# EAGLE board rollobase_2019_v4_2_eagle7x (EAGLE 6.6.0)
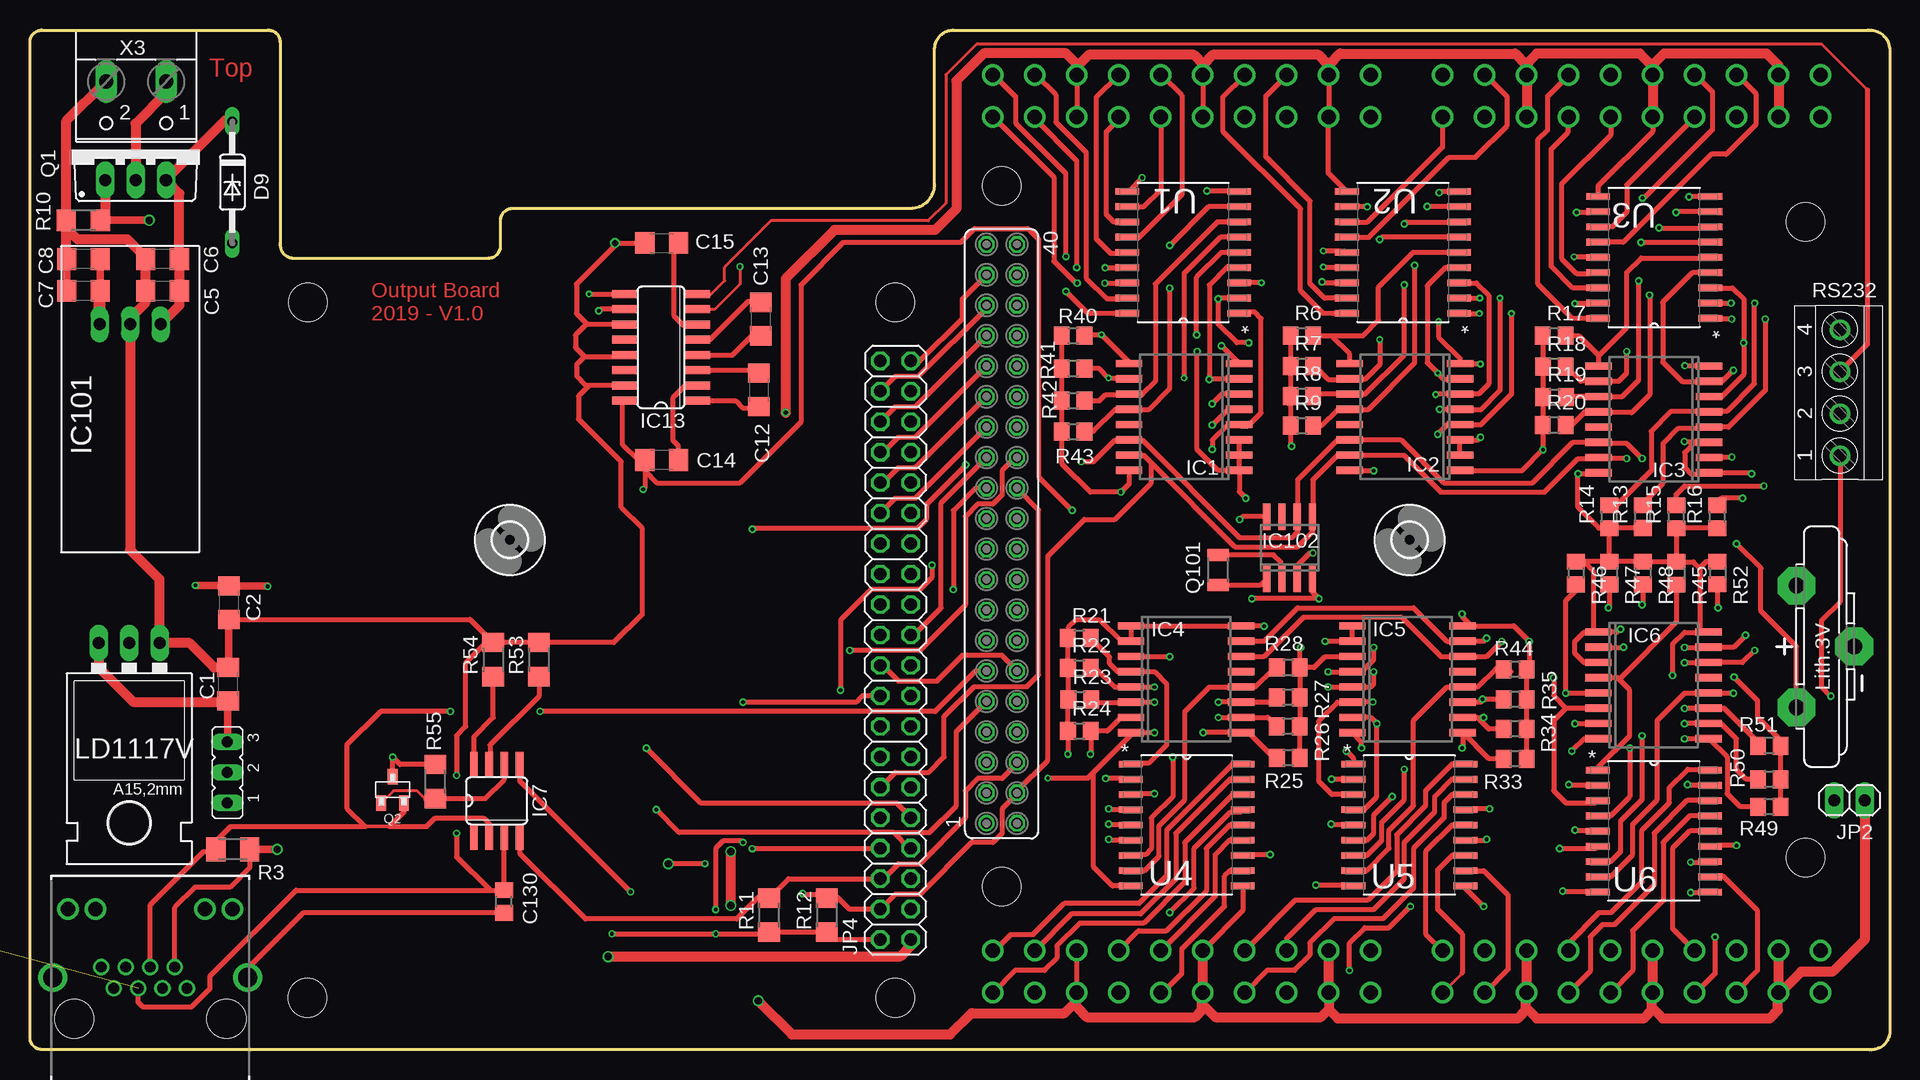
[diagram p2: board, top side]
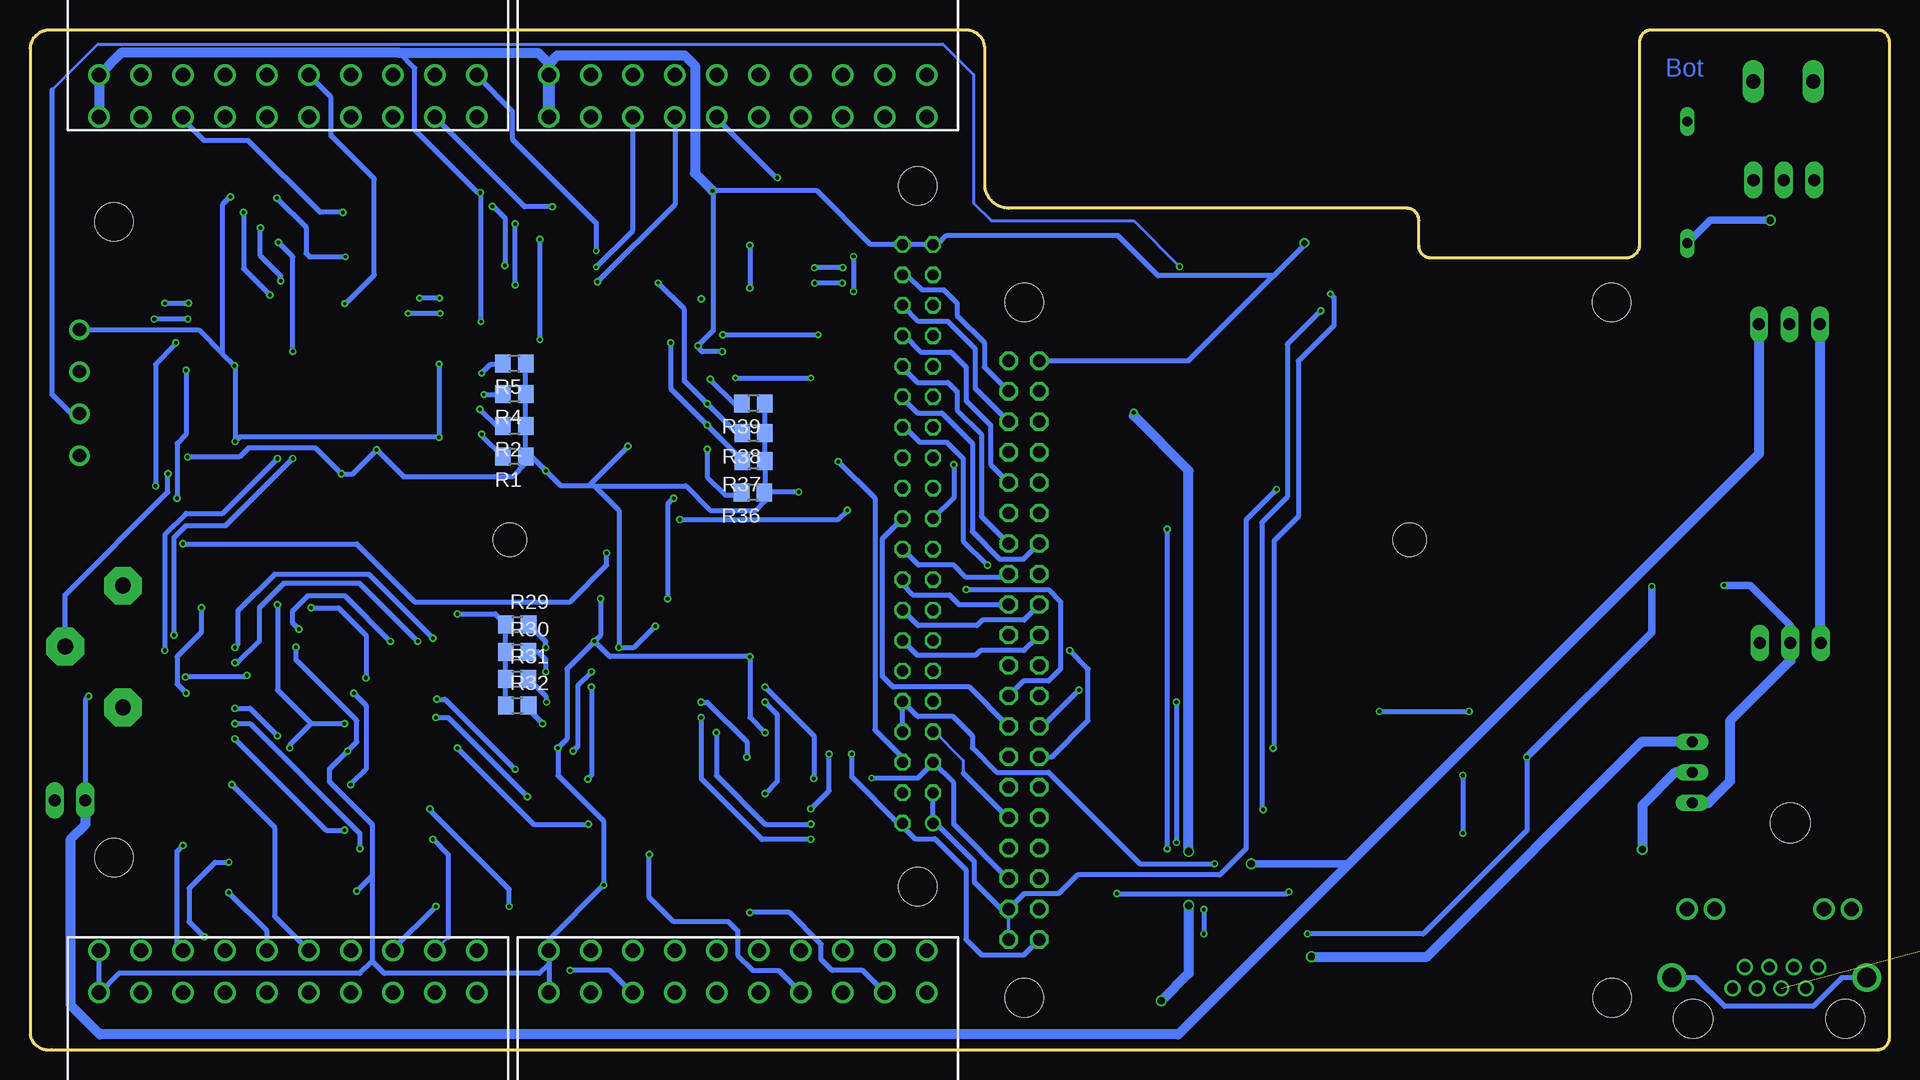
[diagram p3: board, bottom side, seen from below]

Size 155 x 85.03 mm. Coordinates in mm from the lower left corner, seen from the top.
Outline: 153.2,0.02 1,0.02 arc-90 0,1.02 0,84.02 arc-90 1,85.02 19.85,85.02 arc-90 20.85,84.02 20.85,67.27 arc90 21.85,66.02 38.23,66.02 arc90 39.23,67.02 39.23,69.17 arc-90 40.23,70.17 73.42,70.17 arc90 75.42,72.17 75.42,83.52 arc-90 77.02,85.02 153.2,85.02 arc-90 155,83.52 155,1.29 arc-90 153.2,0.02
Copper layers (1*16): Top 0.035mm / dielectric 1.6mm / Bottom 0.035mm
Design rules "JLCPCB_2-layer_PCB_eagle_rule": minimum track width 3.5mil, minimum drill 0.2mm, track to track 6mil, track to pad 6mil, pad to pad 6mil, via to via 8mil, smd to smd 0mil, copper to edge 20mil, drill to drill 10mil, minimum pad ring 6mil, minimum via ring 6mil, stop-mask expansion 0mil, vias tented up to drill 100mil, thermal gap 10mil
Net classes: 0 default: clearance 0.203 mm; 1 signal: width 0.406 mm, drill 0.254 mm, clearance 0.203 mm
Holes 3.2 mm at 23.16,62.33 72.11,62.33 72.14,4.34 81,72.02 81,13.62 148.02,16.02 23.13,4.34 148.02,69.02

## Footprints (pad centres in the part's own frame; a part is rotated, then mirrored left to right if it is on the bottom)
CR2032V = drill 1.321 pad 3.15 octagon: + -2.54,-5.08; +@1 -2.54,5.08; - 2.286,0
C1206 = smd 1.6 x 1.8: 1 -1.4,0; 2 1.4,0
R0805 = smd 1.3 x 1.5: 1 -0.95,0; 2 0.95,0
DO35Z10 = drill 0.813 long: A 5.08,0; C -5.08,0
SO16W = smd 0.6 x 2.2: 1 -4.445,-4.6; 2 -3.175,-4.6; 3 -1.905,-4.6; 4 -0.635,-4.6; 5 0.635,-4.6; 6 1.905,-4.6; 7 3.175,-4.6; 8 4.445,-4.6; 9 4.445,4.6; 10 3.175,4.6; 11 1.905,4.6; 12 0.635,4.6; 13 -0.635,4.6; 14 -1.905,4.6; 15 -3.175,4.6; 16 -4.445,4.6
SO08 = smd 0.66 x 2.032: 1 -1.905,-3.073; 2 -0.635,-3.073; 3 0.635,-3.073; 4 1.905,-3.073; 5 1.905,3.073; 6 0.635,3.073; 7 -0.635,3.073; 8 -1.905,3.073
SO16 = smd 0.66 x 2.032: 1 -4.445,-3.073; 2 -3.175,-3.073; 3 -1.905,-3.073; 4 -0.635,-3.073; 5 0.635,-3.073; 6 1.905,-3.073; 7 3.175,-3.073; 8 4.445,-3.073; 9 4.445,3.073; 10 3.175,3.073; 11 1.905,3.073; 12 0.635,3.073; 13 -0.635,3.073; 14 -1.905,3.073; 15 -3.175,3.073; 16 -4.445,3.073
SIP3 = drill 1 long: 1 -2.54,0; 2 0,0; 3 2.54,0
SO08' = smd 0.6 x 2.2: 1 -1.905,-2.6; 2 -0.635,-2.6; 3 0.635,-2.6; 4 1.905,-2.6; 5 1.905,2.6; 6 0.635,2.6; 7 -0.635,2.6; 8 -1.905,2.6
0569564 = drill 0.9: 1 -4.445,6.35; 2 -3.175,8.89; 3 -1.905,6.35; 4 -0.635,8.89; 5 0.635,6.35; 6 1.905,8.89; 7 3.175,6.35; 8 4.445,8.89 | drill 1.2: A1 -6.295,-4.32; A2 3.835,-4.32; C1 -3.755,-2.79; C2 6.375,-2.79 | drill 1.6: S1 -7.745,3.05; S2 7.745,3.05 | hole 3.25: -5.715,0; 5.715,0
0569564' = drill 0.9: 1 3.06,-0.89; 2 2.04,0.89; 3 1.02,-0.89; 4 0,0.89; 5 -1.02,-0.89; 6 -2.04,0.89; 7 -3.06,-0.89; 8 -4.08,0.89 | drill 1.2: A1 -6.86,5.71; A2 4.57,5.71; C1 -4.57,5.71; C2 6.86,5.71 | drill 1.6: S1 8.125,0; S2 -8.125,0 | hole 3.25: -6.35,-3.43; 6.35,-3.43
FE20-2 = drill 0.914: 1 -24.13,1.27 | drill 0.914 octagon: 2 -24.13,-1.27; 3 -21.59,1.27; 4 -21.59,-1.27; 5 -19.05,1.27; 6 -19.05,-1.27; 7 -16.51,1.27; 8 -16.51,-1.27; 9 -13.97,1.27; 10 -13.97,-1.27; 11 -11.43,1.27; 12 -11.43,-1.27; 13 -8.89,1.27; 14 -8.89,-1.27; 15 -6.35,1.27; 16 -6.35,-1.27; 17 -3.81,1.27; 18 -3.81,-1.27; 19 -1.27,1.27; 20 -1.27,-1.27; 21 1.27,1.27; 22 1.27,-1.27; 23 3.81,1.27; 24 3.81,-1.27; 25 6.35,1.27; 26 6.35,-1.27; 27 8.89,1.27; 28 8.89,-1.27; 29 11.43,1.27; 30 11.43,-1.27; 31 13.97,1.27; 32 13.97,-1.27; 33 16.51,1.27; 34 16.51,-1.27; 35 19.05,1.27; 36 19.05,-1.27; 37 21.59,1.27; 38 21.59,-1.27; 39 24.13,1.27; 40 24.13,-1.27
1X02 = drill 1.016 long: 1 -1.27,0; 2 1.27,0
2X20 = drill 1.016 octagon: 1 -24.13,-1.27; 2 -24.13,1.27; 3 -21.59,-1.27; 4 -21.59,1.27; 5 -19.05,-1.27; 6 -19.05,1.27; 7 -16.51,-1.27; 8 -16.51,1.27; 9 -13.97,-1.27; 10 -13.97,1.27; 11 -11.43,-1.27; 12 -11.43,1.27; 13 -8.89,-1.27; 14 -8.89,1.27; 15 -6.35,-1.27; 16 -6.35,1.27; 17 -3.81,-1.27; 18 -3.81,1.27; 19 -1.27,-1.27; 20 -1.27,1.27; 21 1.27,-1.27; 22 1.27,1.27; 23 3.81,-1.27; 24 3.81,1.27; 25 6.35,-1.27; 26 6.35,1.27; 27 8.89,-1.27; 28 8.89,1.27; 29 11.43,-1.27; 30 11.43,1.27; 31 13.97,-1.27; 32 13.97,1.27; 33 16.51,-1.27; 34 16.51,1.27; 35 19.05,-1.27; 36 19.05,1.27; 37 21.59,-1.27; 38 21.59,1.27; 39 24.13,-1.27; 40 24.13,1.27
78XXL = drill 1.016 long: GND 0,-3.81; IN -2.54,-3.81; OUT 2.54,-3.81 | hole 3.302: 0,11.176
JP2 = drill 0.914 long: 1 -2.54,0; 2 0,0; 3 2.54,0
713-1425 = drill 1.2: 1 -15.75,-1.75; 2 -15.75,1.75; 3 -12.25,-1.75; 4 -12.25,1.75; 5 -8.75,-1.75; 6 -8.75,1.75; 7 -5.25,-1.75; 8 -5.25,1.75; 9 -1.75,-1.75; 10 -1.75,1.75; 11 1.75,-1.75; 12 1.75,1.75; 13 5.25,-1.75; 14 5.25,1.75; 15 8.75,-1.75; 16 8.75,1.75; 17 12.25,-1.75; 18 12.25,1.75; 19 15.75,-1.75; 20 15.75,1.75
TO220BV = drill 1.016 long: D 0,-2.54; G -2.54,-2.54; S 2.54,-2.54
SOT23 = smd 1.3 x 0.9: 1 -1.1,0.95; 2 -1.1,-0.95; 3 1.1,0
QSMD = smd 1 x 1.8: 1 -1.25,0; 2 1.25,0
M1206 = smd 1.6 x 2: 1 -1.4,0; 2 1.4,0
R1206 = smd 1.6 x 1.803: 1 -1.422,0; 2 1.422,0
TERMINAL-BLOCK-4-PIN-3.5MM-ROUND-PAD = drill 1.1 pad 1.7: 1 -5.25,-0.1; 2 -1.75,-0.1; 3 1.75,-0.1; 4 5.25,-0.1
TIULN2803ADW_SOIC127P1030X265-18N = smd 1.981 x 0.559: 1 -4.674,5.08; 2 -4.674,3.81; 3 -4.674,2.54; 4 -4.674,1.27; 5 -4.674,0; 6 -4.674,-1.27; 7 -4.674,-2.54; 8 -4.674,-3.81; 9 -4.674,-5.08; 10 4.674,-5.08; 11 4.674,-3.81; 12 4.674,-2.54; 13 4.674,-1.27; 14 4.674,0; 15 4.674,1.27; 16 4.674,2.54; 17 4.674,3.81; 18 4.674,5.08
2,8 = hole 2.8: 0,0
RJ45-TRAFO-L = drill 1: 1 -4.445,6.35; 2 -3.175,8.89; 3 -1.905,6.35; 4 -0.635,8.89; 5 0.635,6.35; 6 1.905,8.89; 7 3.175,6.35; 8 4.445,8.89 | drill 1.6: GND1 -7.62,2.54; GND2 7.62,2.54 | drill 1.1: LEDG+ -6.35,-5.08; LEDG- -3.81,-5.08; LEDY+ 3.81,-5.08; LEDY- 6.35,-5.08 | hole 3.2: -5.08,0; 5.08,0
W237-102 = drill 1.194 long: 1 -2.5,-1.27; 2 2.5,-1.27

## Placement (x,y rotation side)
BAT  CR2032V  [CR2032V]  149.79,33.62 0 top
C1  1uF  [C1206]  16.52,30.48 90 top
C2  1uF  [C1206]  16.57,37.29 270 top
C5  1uF  [C1206]  11.05,63.27 180 top
C6  1uF  [C1206]  11.05,65.92 180 top
C7  1uF  [C1206]  4.45,63.27 180 top
C8  1uF  [C1206]  4.45,65.92 180 top
C12  1µF  [C1206]  60.75,55.02 270 top
C13  1µF  [C1206]  60.9,60.92 270 top
C14  1µF  [C1206]  52.65,49.17 180 top
C15  1µF  [C1206]  52.65,67.27 0 top
C130  1nF  [R0805]  39.51,12.37 90 top
D9  ZPD  [DO35Z10]  16.86,72.33 270 top
IC1  PCF8574T  [SO16W]  96.21,52.77 90 top
IC2  PCF8574T  [SO16W]  114.6,52.77 90 top
IC3  PCF8574T  [SO16W]  135.35,52.57 90 top
IC4  PCF8574T  [SO16W]  96.37,30.9 270 top
IC5  PCF8574T  [SO16W]  114.83,30.9 270 top
IC6  PCF8574T  [SO16W]  135.33,30.39 270 top
IC7  DS2482-100S  [SO08]  38.91,20.77 0 top
IC13  MAX3232CSE  [SO16]  52.6,58.57 90 top
IC101  R-78B5.0_SIP3  [SIP3]  8.34,60.49 180 top
IC102  DS1307_SO8  [SO08']  104.99,41.86 0 top
J1  0569564-2  [0569564]  not placed on the board
J103  0569564-  [0569564']  10.03,6.02 0 top
JP1  jp1  [FE20-2]  81,43.02 90 top
JP2  0  [1X02]  151.66,20.8 0 top
JP4  0  [2X20]  72.15,33.32 90 top
LD1117V  V_REG_LD1117VXX  [78XXL]  8.26,30.11 180 top
OW  0  [JP2]  16.45,23.12 90 top
P13  713-1430  [713-1425]  96,79.52 180 bottom
P14  713-1430  [713-1425]  133.5,79.51 180 bottom
P15  713-1430  [713-1425]  96,6.52 0 bottom
P16  713-1430  [713-1425]  133.5,6.52 0 bottom
Q1  IRF9530  [TO220BV]  8.8,75.06 0 top
Q2  TSM 3401 SOT-23  [SOT23]  30.23,21.69 90 top
Q101  32.768KHZ_SMD  [QSMD]  99.04,40.01 270 top
R1  1k  [R0805]  114.63,49.46 180 bottom
R2  1k  [R0805]  114.63,51.99 180 bottom
R3  2k2  [M1206]  16.9,16.72 0 top
R4  1k  [R0805]  114.63,54.68 180 bottom
R5  1k  [R0805]  114.63,57.21 180 bottom
R6  1k  [R0805]  106.02,59.55 0 top
R7  1k  [R0805]  106.02,57.02 0 top
R8  1k  [R0805]  106.02,54.49 0 top
R9  1k  [R0805]  106.02,52.06 0 top
R10  100K  [R1206]  4.45,69.16 0 top
R11  1k  [R1206]  61.6,11.24 90 top
R12  1k  [R1206]  66.41,11.24 90 top
R13  1k  [R0805]  134.44,44.46 90 top
R14  1k  [R0805]  131.65,44.45 90 top
R15  1k  [R0805]  137.23,44.45 90 top
R16  1k  [R0805]  140.65,44.45 90 top
R17  1k  [R0805]  127.04,59.54 0 top
R18  1k  [R0805]  127.06,56.98 0 top
R19  1k  [R0805]  127.09,54.43 0 top
R20  1k  [R0805]  127.04,52.1 0 top
R21  1k  [R0805]  87.46,34.33 0 top
R22  1k  [R0805]  87.47,31.85 0 top
R23  1k  [R0805]  87.51,29.21 0 top
R24  1k  [R0805]  87.47,26.58 0 top
R25  1k  [R0805]  104.89,24.35 180 top
R26  1k  [R0805]  104.88,26.97 180 top
R27  1k  [R0805]  104.89,29.38 180 top
R28  1k  [R0805]  104.89,31.87 180 top
R29  1k  [R0805]  114.39,35.47 0 bottom
R30  1k  [R0805]  114.39,33.18 0 bottom
R31  1k  [R0805]  114.4,30.92 0 bottom
R32  1k  [R0805]  114.39,28.71 0 bottom
R33  1k  [R0805]  123.79,24.27 180 top
R34  1k  [R0805]  123.79,26.76 180 top
R35  1k  [R0805]  123.79,29.23 180 top
R36  1k  [R0805]  94.74,46.46 180 bottom
R37  1k  [R0805]  94.69,49.09 180 bottom
R38  1k  [R0805]  94.69,51.41 180 bottom
R39  1k  [R0805]  94.72,53.9 180 bottom
R40  1k  [R0805]  86.95,59.55 0 top
R41  1k  [R0805]  86.95,56.82 0 top
R42  1k  [R0805]  86.95,54.13 0 top
R43  1k  [R0805]  86.95,51.55 0 top
R44  1k  [R0805]  123.79,31.71 180 top
R45  1k  [R0805]  137.24,39.73 270 top
R46  1k  [R0805]  128.86,39.75 270 top
R47  1k  [R0805]  131.65,39.75 270 top
R48  1k  [R0805]  134.44,39.75 270 top
R49  1k  [R0805]  144.98,20.27 180 top
R50  1k  [R0805]  144.98,22.55 180 top
R51  1k  [R0805]  144.98,25.35 180 top
R52  1k  [R0805]  140.66,39.76 270 top
R53  0R  [R1206]  42.42,32.53 90 top
R54  0R  [R1206]  38.61,32.53 90 top
R55  0R  [R1206]  33.78,22.37 270 top
RS232  TERMINAL-BLOCK-3.5MM -- RND 205-00102  [TERMINAL-BLOCK-4-PIN-3.5MM-ROUND-PAD]  150.77,54.79 90 top
U1  TIULN2803ADW_ULN2803ADW  [TIULN2803ADW_SOIC127P1030X265-18N]  96.12,66.48 180 top
U2  TIULN2803ADW_ULN2803ADW  [TIULN2803ADW_SOIC127P1030X265-18N]  114.45,66.48 180 top
U3  TIULN2803ADW_ULN2803ADW  [TIULN2803ADW_SOIC127P1030X265-18N]  135.38,66.07 180 top
U4  TIULN2803ADW_ULN2803ADW  [TIULN2803ADW_SOIC127P1030X265-18N]  96.42,18.75 0 top
U5  TIULN2803ADW_ULN2803ADW  [TIULN2803ADW_SOIC127P1030X265-18N]  114.97,18.75 0 top
U6  TIULN2803ADW_ULN2803ADW  [TIULN2803ADW_SOIC127P1030X265-18N]  135.37,18.24 0 top
U$1  [2,8]  40,42.52 0 top
U$2  [2,8]  115,42.52 0 top
U$3  RJ45-TRAFO-L  [RJ45-TRAFO-L]  not placed on the board
U$4  [WAGO288-001]  40.14,42.52 270 top
X3  VERSORGUNG  [W237-102]  8.85,79.46 180 top

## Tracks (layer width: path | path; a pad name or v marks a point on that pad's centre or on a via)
$N5555
  Top 0.406: J103.S1 18.15,6.79 22.79,11.42 C130.1
  Bottom 0.406: J103.S2 3.96,6.02 6.36,3.62 13.75,3.62 16.15,6.02 J103.S1
+3V3  (via drill 0.3)
  Top 0.254: 16.53,38.72 C2.1 | 67,9.19 67,9.23 | 61.46,9.67 R11.1 | v19.81,38.63 19.75,38.69
  Top 0.406: JP4.2 67,9.19 | 129.5,40.7 130.3,39.9 130.3,34.98 130.46,34.82 | IC1.16 91.61,47.18 v90.93,46.5 88.39,46.5 86,48.9 R43.1 R42.1 R41.1 R40.1 | R6.1 R7.1 R8.1 | R8.1 105.07,54.04 104.9,53.87 104.9,54.32 R8.1 | R8.1 R9.1 105.07,50.4 v105.16,50.31 | IC2.16 111.98,48.32 v112.01,48.28 | R17.1 126.09,57 R18.1 126.11,54.45 R19.1 126.14,52.15 | v105.92,33.55 105.84,33.47 R28.1 | v102.87,35.33 100.98,35.33 IC4.16 IC4.1 IC4.2 90.92,34.07 89.15,35.84 87.17,35.84 86.54,35.2 86.54,34.36 R21.1 86.52,34.32 R22.1 86.56,31.8 R23.1 86.52,29.16 R24.1 v86.52,24.67 v86.51,24.66 | R49.1 R50.1 R51.1 145.93,25.8 144.02,27.71 144.02,29.11 v142.04,31.09 | 138.94,34.82 137.92,34.82 136.91,33.8 v136.91,31.21 | 138.94,34.82 139.92,34.82 IC6.16 | R45.1 134.46,40.68 R48.1 R47.1 | R47.1 129.5,40.7 | R45.1 138.66,40.68 139.19,40.15 | 139.19,40.15 139.19,35.07 138.94,34.82 | 120.14,35.34 123.68,35.34 v124.97,34.06 124.97,31.94 R44.1 R35.1 R34.1 R33.1 | v132.59,35.07 132.51,35.07 132.27,34.83 IC6.1 130.48,34.83 130.46,34.82 | R28.1 107.03,31.87 107.95,32.79 110.21,32.79 IC5.3 | IC5.16 120.14,35.34 | 126.14,52.15 126.14,50.06 v126.11,50.04 124.4,48.32 IC2.1 | 126.14,52.15 R20.1 | 129.5,40.7 R46.1 | R16.1 R15.1 R45.1 | R47.1 R14.1 | R13.1 R14.1 | R14.1 130.76,43.51 129.03,45.23 v129.03,48.03 130.66,48.03 IC3.16 | Q2.3 v30.23,24.41 30.84,23.8 R55.1 | R28.1 R27.1 105.84,26.97 R26.1 105.83,24.36 R25.1 | R52.1 139.74,40.71 139.19,40.15 | v119.38,36.34 119.38,36.1 120.14,35.34 | IC6.3 130.72,32.28 129.54,32.28 128.78,33.04 128.78,34.06 129.54,34.82 130.46,34.82 | R11.1 R12.1 67,9.23 | JP4.18 69.37,29.51 68.83,28.98 v59.44,28.98
  Top 0.406: v59.44,17.29 59.31,17.42 57.78,17.42 57.15,16.79 v57.15,11.71 | 61.46,9.67 v57.15,9.67 v48.51,9.67 | IC3.2 141.82,49.39 v141.86,49.43
  Top 0.61: v13.8,38.72 16.53,38.72 | 19.75,38.69 C2.1
  Bottom 0.406: JP4.2 72.15,7.92 75.7,7.92 77,9.22 77,15.02 79.58,17.6 81.24,17.6 82.27,18.63 JP1.2 82.34,18.82 82.55,18.82 86.51,22.78 v86.51,24.66 | v141.86,49.43 137.54,49.43 136.78,50.19 131.19,50.19 v129.03,48.03 128.11,48.03 v126.11,50.02 v126.11,50.04 126.09,50.04 123.83,47.77 114.81,47.77 113.68,48.9 R1.1 | R36.1 93.74,46.51 R37.1 R38.1 93.74,53.88 R39.1 | R1.1 113.59,49.55 113.28,49.55 v112.01,48.28 110.74,47.01 108.46,47.01 | R1.1 R2.1 R4.1 R5.1 | 107.95,47.01 108.46,47.01 | v105.16,50.31 108.46,47.01 | v102.87,35.33 104.65,33.55 v105.92,33.55 105.9,33.57 105.9,44.96 107.95,47.01 | v136.91,31.21 136.98,31.14 141.99,31.14 v142.04,31.09 | v132.59,35.07 133.1,35.58 133.1,36.6 131.83,37.87 128.78,37.87 v124.97,34.06 | v119.38,36.34 116.21,36.34 R29.1 R30.1 R31.1 115.34,30.92 R32.1 | v90.93,46.5 93.75,46.5 R36.1 | R36.1 93.73,46.4 93.73,45.74 94.49,44.98 98.3,44.98 100.33,47.01 107.95,47.01 | v59.44,28.98 v59.44,17.29 | v57.15,11.71 v57.15,9.67 | v30.23,24.41 30.23,18.31 38.86,9.67 v48.51,9.67
  Bottom 0.61: v13.8,38.72 11.59,38.72 8.26,35.4 LD1117V.GND | v19.81,38.63 19.81,34.82 v30.23,24.41
  Bottom 0.813: OW.1 15.1,20.58 13.3,22.38 13.3,27.42 8.26,32.46 LD1117V.GND
+5V  (via drill 0.3, 0.6)
  Top 0.254: 51.25,48.28 C14.2 50.67,49.17 | 49.4,54 IC13.16 | 16.46,29.02 C1.1
  Top 0.406: v51.1,46.72 51.25,46.87 51.25,48.28 52.27,47.27 59.18,47.27 64.26,52.35 64.26,63.78 67.82,67.33 77.6,67.33 78.74,68.48 83.19,68.48 84.07,67.59 84.07,47.77 v86.87,44.98 | 50.67,49.17 49.4,50.44 49.4,54 | IC102.8 101.08,44.46 v100.84,44.22
  Top 0.61: C8.1 C7.1 | 73.41,9.18 JP4.1 | 16.46,29.02 OW.3
  Top 0.813: LD1117V.OUT 5.72,31.89 8.59,29.02 16.46,29.02 | v48.19,7.77 72.52,7.77 73.41,8.66 73.41,9.18
  Top 1.016: IC101.3 5.8,63.22 C7.1
  Bottom 0.254: JP4.1
  Bottom 0.305: JP4.3 JP4.1
  Bottom 0.406: JP4.3 74.03,11.72 76.3,13.99 76.3,15.73 79.46,18.89 JP1.1 JP1.3 | v51.1,46.72 53.64,44.18 53.64,16.77 55.83,14.58 67.71,14.58 69.26,13.02 72.13,13.02 JP4.3 | v86.87,44.98 87.63,44.22 v100.84,44.22
  Bottom 0.61: 5.8,34 LD1117V.OUT | IC101.3 | 20.59,25.66 20.63,25.7
  Bottom 0.813: IC101.3 5.8,34 | v48.19,7.77 38.56,7.77 20.63,25.7 | OW.3 20.59,25.66
+12V  (via drill 0.3, 0.6)
  Top 0.254: C6.1 12.45,65.98
  Top 0.406: v56.26,15.52 v53.21,15.52 | v150.11,29.49 149.35,30.25 149.35,35.84 150.88,37.36 RS232.1
  Top 0.61: 11.34,72.58 Q1.S 11.34,72.5 | 16.26,77.49 16.78,77.49
  Top 0.813: 11.34,72.58 16.26,77.49 | 16.78,77.49 D9.C | 11.34,72.5 12.45,71.4 12.45,65.98 | C6.1 C5.1 12.45,62.06 IC101.1
  Bottom 0.406: v56.26,15.52 62.48,15.52 70.1,23.14 74.42,23.14 76.45,25.17 76.45,26.18 78.05,27.78 81,27.78 JP1.10 JP1.8 | JP2.1 150.39,29.21 v150.11,29.49
  Bottom 0.61: 150.37,20.78 JP2.1 | 45.58,14.99 45.57,14.99 | 45.05,15.52 v53.21,15.52
  Bottom 0.813: 150.37,20.78 150.37,18.82 151.6,17.59 151.6,3.72 149.17,1.29 59.28,1.29 45.58,14.99 | 45.57,14.99 45.05,15.52 10.88,49.69 IC101.1
+12VIN
  Top 0.61: X3.1 11.35,79.78
  Top 0.813: 11.35,79.78 8.8,77.23 Q1.D
CE0
  Bottom 0.406: JP4.23 77.56,37.13 78.38,37.94 81.43,37.94 82.27,38.78 JP1.18
CE1
  Bottom 0.406: JP4.25 73.42,39.63 73.66,39.39 76.96,39.39 77.98,40.41 80.93,40.41 JP1.20
GND  (via drill 0.25, 0.3, 0.5)  (1 unrouted)
  Top 0.254: v48.77,67.27 48.77,67.06 | C7.2 3.05,63.15 | C5.2 9.63,63.27 9.59,63.31 | C8.2 3,65.92 | 38.01,33.96 R54.2
  Top 0.305: 38.35,13.32 C130.2 39.27,13.32 39.26,13.31 | 39.51,17.66 IC7.3
  Top 0.406: 38.35,13.32 35.56,16.11 v35.56,18.06 | C130.2 39.51,17.66 | v98.11,71.62 100.74,71.62 U1.9 | IC1.1 IC1.2 IC1.3 | v117.41,60.71 117.41,59.44 119.19,57.66 119.2,57.66 IC2.8 119.24,57.17 v120.9,57.17 | U3.9 138.32,71.15 v138.3,71.12 | 48.77,67.06 45.56,63.85 45.56,61.39 46.48,60.47 IC13.11 46.36,60.48 45.47,59.59 45.47,58.57 46.23,57.81 | v137.9,50.72 137.96,50.66 IC3.3 138.78,50.66 137.92,49.81 137.92,48.54 138.43,48.03 139.86,48.03 IC3.1 143.42,48.12 v143.51,48.03 | IC6.2 v132.83,33.56 | U6.9 127.83,13.16 v127.76,13.23 | v48.77,67.27 C15.1 | IC1.8 v99.31,58.7 | v97.28,58.21 97.28,50.06 99.02,48.32 IC1.1 | IC2.2 IC2.3 120.69,50.86 v120.9,51.08 | v107.19,13.74 110.23,13.74 U5.9 | IC6.8 129.55,25.94 v128.52,24.91 | U4.9 90.24,13.67 88.65,15.26 88.65,23.14 | IC5.1 IC5.2 107.96,34.07 v107.95,34.06 | v111,25.17 111,25.68 IC5.8 | IC4.3 91.81,32.8 91.82,32.79 v95,32.79 | v93.73,26.44 91.78,26.44 | 91.78,26.44 IC4.8 | IC3.8 137.98,57.01 v137.95,57.05 | 91.78,26.44 91.78,26.27 88.65,23.14 | IC102.4 106.89,38.16 v107.44,37.61 v101.85,37.61 | IC1.1 100.81,46.54 v101.35,46 | v35.56,22.88 35.56,26.18 36.32,26.95 36.32,32.26 38.01,33.96 | v84.84,22.65 88.16,22.65 88.65,23.14 | 39.26,13.31 22.18,13.31 14.99,6.12 14.99,5.1 13.46,3.58 9.4,3.58 9.01,3.97 J103.5 | U2.9 117.55,71.56 v117.45,71.47 | C2.2 36.68,35.89 R54.2 R53.2 48.67,33.96 51.05,36.34 51.05,43.46 49.28,45.23 49.28,49.04 45.72,52.6 45.72,54.51 46.61,55.4 IC13.15 46.35,55.4 45.59,56.16 45.59,57.17 46.23,57.81 | 46.23,57.81 49.4,57.81 IC13.13
  Top 0.61: X3.2 6.3,80.73 | R10.1 3,69.13 3,68.56 | 3.05,63.15 C8.2 | C2.2 16.57,31.93 C1.2 | C6.2 9.65,66.05
  Top 0.813: 3,65.92 3,68.56 4,67.56 8.13,67.56 9.65,66.05 | C5.2 C6.2 | R10.1 3.03,77.46 6.3,80.73 | 9.59,63.31 9.59,62.25 8.34,61 IC101.2 8.34,41.69 10.8,39.22 LD1117V.IN 13.3,33.92 15.34,31.88 C1.2
  Bottom 0.254: 111.75,7.14 P15.2 111.75,9.18 | v98.11,71.62 98.04,71.56 | JP1.5 79.73,23.92 | 51.31,64.54 51.35,64.54 | 73.49,14.27 JP4.5
  Bottom 0.406: P16.2 P16.1 149.25,4.72 147.6,6.37 127.51,6.37 126.49,7.39 | v98.11,71.62 89.4,71.62 84.93,67.15 JP1.40 JP1.39 79.35,67.15 78.59,67.91 64.34,67.91 60.96,64.54 51.35,64.54 58.44,57.45 JP4.40 | v117.41,60.71 117.45,60.75 v117.45,71.47 117.67,71.47 122.94,76.73 122.94,81.84 124.21,83.11 | v138.3,71.12 138.96,70.46 138.96,58.05 | 73.49,14.27 78,18.78 78,22.24 JP1.5 | 126.49,14.5 126.49,7.39 | P15.2 P15.1 | 111.75,7.14 112.52,6.37 125.48,6.37 126.49,7.39 | 111.75,9.18 v107.19,13.74 107.19,19.07 111,22.88 v111,25.17 110.24,25.93 110.24,31.77 v107.95,34.06 | v132.83,33.56 132.84,33.55 132.84,32.53 127.76,27.45 127.76,25.68 v128.52,24.91 130.05,23.39 130.05,22.37 126.49,18.82 126.49,14.5 | 79.73,23.92 81,22.65 v84.84,22.65 | v93.73,26.44 95,27.71 v95,32.79 106.68,32.79 v107.95,34.06 | v120.9,57.17 v120.9,51.08 137.54,51.08 v137.9,50.72 137.9,56.99 v137.95,57.05 138.96,58.05 | v35.56,22.88 v35.56,18.06 | 126.49,14.5 v127.76,13.23 | v143.51,48.03 143.51,46.5 152.07,37.94 BAT.- | RS232.4 140.94,60.04 138.96,58.05 | v107.44,37.61 107.44,34.57 v107.95,34.06 | v48.77,67.27 48.77,67.08 51.31,64.54 | v101.35,46 101.85,45.49 v101.85,37.61 | 98.04,71.56 98.04,59.97 v99.31,58.7 99.31,58.57 98.96,58.21 v97.28,58.21
  Bottom 0.813: P14.20 P14.19 147.4,83.11 124.21,83.11 112.65,83.11 111.75,82.21 111.05,82.91 100.42,82.91 99.57,82.06 99.57,73.08 v98.11,71.62
  Bottom 1.016: P13.20 P13.19 111.75,82.21
GPCLK0  (via drill 0.3)
  Top 0.254: JP4.8 70.83,16.76
  Top 0.406: v78,48.77 74.75,45.52 74.75,44.27 74,43.52 60.34,43.52 v60.22,43.4 | 70.83,16.76 v60.22,16.76
  Bottom 0.406: JP1.21 78,46.02 v78,48.77 | v60.22,43.4 v60.22,16.76
GPIO5
  Top 0.406: JP4.30 70.89,44.75 72.14,46 73.81,46 JP1.27
GPIO6
  Top 0.406: JP4.32 71.15,47.29 72.39,48.54 73.81,48.54 JP1.29
GPIO12
  Bottom 0.406: JP1.34 82.12,59.53 80.77,58.19 78.23,58.19 76.96,56.92 76.96,54.12 74.93,52.09 74.93,48.8 JP4.31
GPIO13
  Top 0.406: JP4.34 71.15,49.83 72.39,51.08 73.81,51.08 JP1.31
GPIO16
  Bottom 0.406: JP4.35 73.43,52.37 76.2,55.14 76.2,58.44 78.49,60.73 80.93,60.73 JP1.36
GPIO18
  Top 0.254: JP4.12 70.89,21.89
  Top 0.406: 70.89,21.89 72.14,23.14 74.93,23.14 76.2,24.41 76.2,27.78 78.72,30.3 83.11,30.3 84.07,31.26 84.07,45.03 JP1.24
GPIO19
  Top 0.406: JP4.36 70.89,52.37 72.14,53.62 73.81,53.62 JP1.33
GPIO20
  Bottom 0.406: JP1.38 81.89,64.61 80.64,63.37 78.84,63.37 77.72,62.25 77.72,61.24 75.44,58.95 75.44,56.93 JP4.37
GPIO21
  Top 0.406: JP1.37 77.72,62.61 77.72,60.98 74.19,57.45 JP4.39
GPIO22  (via drill 0.3)
  Top 0.406: v75.18,40.41 75.18,39.39 74.17,38.38 70.1,38.38 67.56,35.84 v67.56,29.99
  Bottom 0.406: JP1.28 82.12,51.91 80.87,50.67 78.59,50.67 77.22,49.3 77.22,42.44 v75.18,40.41 | v67.56,29.99 70.61,26.95 70.85,26.95 JP4.16
GPIO23
  Bottom 0.406: JP4.15 73.43,26.97 76.71,30.25 83.06,30.25 83.95,31.14 83.95,42.62 JP1.22
GPIO24  (via drill 0.3)
  Top 0.406: JP1.23 78.81,46.83 76.96,44.98 v76.96,38.38
  Bottom 0.406: v76.96,38.38 70.1,38.38 69.09,37.36 69.09,31.77 70.1,30.76 72.18,30.76 JP4.17
GPIO25
  Top 0.406: JP4.21 73.69,34.59 75.95,36.85 75.95,45.59 JP1.25
GPIO26
  Top 0.406: JP4.38 70.89,54.91 72.14,56.16 74.07,56.16 79.73,61.82 JP1.35
GPIO27  (via drill 0.3)
  Top 0.406: JP1.26 82.12,49.37 81.03,48.28 81.03,46.25 80.26,45.49 78.99,45.49 77.98,44.47 77.98,37.11 74.17,33.3 v68.33,33.3
  Bottom 0.406: JP4.14 69.82,24.43 66.8,27.45 66.8,31.77 v68.33,33.3
I2C_SCL  (via drill 0.3)
  Top 0.254: JP4.6 71.15,14.27 | 61.54,12.72 R11.2
  Top 0.406: 110.04,50.82 114.3,50.82 117.86,47.27 125.22,47.27 128.62,50.66 IC3.14 130.84,50.57 133.1,50.57 v134.37,49.3 | 110.04,50.82 IC2.14 | v122.68,34.06 121.43,32.8 IC5.14 119.39,32.77 119.25,32.77 118.75,32.77 118.75,32.79 117.6,32.79 114.3,36.09 106.17,36.09 102.88,32.8 IC4.14 | v137.92,32.28 139.92,32.28 | 139.92,32.28 IC6.14 | 71.15,14.27 72.39,15.52 74.17,15.52 77.98,19.33 77.98,21.61 78.99,22.63 81.03,22.63 82.27,23.87 JP1.6 | v87.63,49.04 88.65,49.04 90.42,50.82 91.57,50.82 IC1.14 91.64,50.82 92.71,50.82 100.84,42.69 105.16,42.69 105.66,43.2 105.66,44.42 IC102.6 105.66,44.5 105.66,47.52 108.97,50.82 110.04,50.82 | 61.54,12.72 60.71,12.72 58.9,10.92 46.3,10.92 40.81,16.4 IC7.4 | R11.2 63.21,14.27 JP4.6 | v143.76,33.3 142.75,32.28 139.92,32.28
  Bottom 0.406: v122.68,34.06 127.51,38.88 133.86,38.88 135.89,36.85 135.89,34.06 137.67,32.28 v137.92,32.28 | JP1.6 82.27,24.38 84.58,26.69 84.58,46 v87.63,49.04 | v143.76,33.3 143.76,42.95 141.99,44.73 138.94,44.73 v134.37,49.3
I2C_SDA  (via drill 0.3)
  Top 0.254: 67.31,12.72 66.47,12.72 R12.2
  Top 0.406: IC7.5 40.81,22.42 v50.06,13.18 | IC6.15 | 130.66,49.3 129.03,49.3 126.24,46.5 117.6,46.5 114.55,49.55 110.04,49.55 IC2.15 109,49.59 106.93,47.52 106.93,44.5 IC102.5 106.93,44.42 106.93,43.2 105.66,41.93 100.46,41.93 93.47,48.92 | 130.66,49.3 IC3.15 | IC1.15 91.64,49.55 92.84,49.55 93.47,48.92 | v121.41,34.31 121.17,34.07 IC5.15 119.41,34.06 118.11,34.06 115.32,36.85 105.66,36.85 102.88,34.07 IC4.15 | v137.92,33.55 139.92,33.55 IC6.15 | 93.47,48.92 93.47,47.27 90.42,44.22 87.88,44.22 84.84,41.17 84.84,24.15 82.27,21.59 JP1.4 82.27,21.33 81.03,20.09 81.03,18.06 80.26,17.29 78.49,17.29 74.17,12.98 72.12,12.98 JP4.4 68.3,11.73 67.31,12.72 | v133.1,49.3 130.66,49.3 | R12.2 66.15,12.91 64.51,12.91 v64.4,13.02 | IC6.15 142,33.56 v143,34.57
  Bottom 0.254: v50.06,13.18 50.21,13.02
  Bottom 0.406: v64.4,13.02 50.21,13.02 | v121.41,34.31 126.75,39.65 134.62,39.65 137.67,36.6 137.67,33.8 v137.92,33.55 | v143,34.57 143,42.69 141.99,43.71 138.68,43.71 v133.1,49.3
IC1_P1  (via drill 0.3)
  Top 0.406: IC1.5 99.86,53.4 v98.55,52.09 | v101.6,58.95 100.58,58.95 99.06,60.47 99.06,62.58 | 99.06,62.58 v99.03,62.61 | U1.2 99.15,62.67 99.06,62.58
  Bottom 0.406: R37.2 95.64,49.18 v98.55,52.09 101.6,55.14 v101.6,58.95
IC1_P2  (via drill 0.25, 0.3)
  Top 0.406: v122.54,62.67 122.54,55 120.9,53.36 119.24,53.36 IC2.5 117.51,53.4 v117.5,53.41 | U2.2 v120.84,62.67 v120.85,62.67
  Bottom 0.406: v120.85,62.67 v122.54,62.67 | R2.2 116.08,51.99 v117.5,53.41
IC1_P3  (via drill 0.25, 0.3)
  Top 0.406: v123.48,61.4 123.48,54.67 120.9,52.09 119.24,52.09 IC2.4 118.15,52.13 v117.35,51.33 | U2.1 v120.81,61.4 v120.82,61.4
  Bottom 0.406: v120.82,61.4 v123.48,61.4 | v117.35,51.33 117.35,51.23 R1.2
IC1_P4  (via drill 0.25)
  Top 0.406: v117.17,54.63 117.21,54.67 IC2.6 119.22,54.68 120.76,54.68 121.59,55.52 121.59,62.92 120.57,63.94 U2.3
  Bottom 0.406: v117.17,54.63 115.62,54.63 R4.2
IC1_P5  (via drill 0.25)
  Top 0.406: U2.4 117.97,65.21 116.47,63.71 116.47,57.29 v117.35,56.41 117.87,55.88 119.15,55.88 IC2.7
  Bottom 0.406: v117.35,56.41 116.59,57.17 115.61,57.17 R5.2
IC1_P6
  Top 0.406: U2.5 119.11,66.47 115.28,66.47 112.4,63.59 112.4,60.82 111.13,59.55 108.46,59.55 | R6.2 108.46,59.55 | IC2.9 110,58 108.46,59.55
IC1_P7  (via drill 0.25, 0.3)
  Top 0.406: U2.6 112.68,67.75 v112.5,67.57 | R7.2 107.09,57.02 108.2,55.9 109.73,55.9 109.97,55.9 | 109.97,55.9 IC2.10 | v112.5,59.22 112.5,57.15 111.25,55.9 109.97,55.9
  Bottom 0.406: v112.5,59.22 112.5,67.54 112.5,67.55 v112.5,67.57
IC1_P8  (via drill 0.3)
  Top 0.406: U2.7 114.72,69.02 v114.55,68.86 | v114.55,63.78 114.55,57.93 111.29,54.67 IC2.11 107.15,54.67 R8.2
  Bottom 0.406: v114.55,63.78 v114.55,68.86
IC1_P9  (via drill 0.3)
  Top 0.406: 100.92,52.02 IC1.4 | 100.92,52.02 99.75,52.02 98.55,50.82 v98.55,50.06 | 100.92,52.02 101.53,52.02 102.62,53.11 102.62,60.98 102.11,61.49 100.89,61.49 U1.1
  Bottom 0.406: v98.55,50.06 98.55,47.77 97.03,46.25 95.9,46.25 R36.2
IC1_P10  (via drill 0.25, 0.3)
  Top 0.406: IC1.6 99.35,54.67 v98.55,53.87 | v102.64,63.95 100.81,63.95 U1.3
  Bottom 0.406: R38.2 95.82,51.58 96.27,51.58 v98.55,53.87 100.46,55.78 100.46,61.75 102.64,63.94 v102.64,63.95
IC1_P11  (via drill 0.3)
  Top 0.406: U1.4 100.71,65.3 99.82,65.3 98.3,63.78 v98.3,55.9 98.33,55.94 IC1.7
  Bottom 0.406: v98.3,55.9 96.27,53.87 95.7,53.87 R39.2
IC1_P12  (via drill 0.25, 0.3)
  Top 0.406: U1.5 99.31,66.48 97.25,64.42 v97.25,59.62 | R40.2 87.97,59.62 v89.31,59.62 91.61,57.33 IC1.9
  Bottom 0.406: v97.25,59.62 v89.31,59.62
IC1_P13  (via drill 0.25)
  Top 0.406: U1.6 99.23,67.75 96.2,64.72 v96.2,56.02 | IC1.10 91.53,56.02 v89.91,56.02 89.15,56.78 88.44,56.78 88.41,56.82 R41.2
  Bottom 0.406: v96.2,56.02 v89.91,56.02
IC1_P14
  Top 0.406: R42.2 89.16,54.13 89.66,54.63 91.57,54.63 IC1.11 91.66,54.62 92.69,54.62 93.8,55.73 93.8,63.85 98.97,69.02 U1.7
IC1_P15  (via drill 0.3)
  Top 0.406: U1.8 98.23,70.29 v95,67.06 | v95,63.51 95,55.14 93.22,53.36 91.64,53.36 IC1.12 90.46,53.4 88.65,51.58 87.94,51.58 R43.2
  Bottom 0.406: v95,63.51 v95,67.06
IC1_P16  (via drill 0.3)
  Top 0.406: U2.8 116.48,70.29 v116.45,70.32 | v115.41,65.41 115.41,57.26 111.51,53.36 110.04,53.36 IC2.12 109.97,53.36 108.97,53.36 107.66,52.06 R9.2
  Bottom 0.406: v116.45,70.32 116.38,70.32 115.41,69.35 v115.41,65.41
IC1_P17  (via drill 0.3)
  Top 0.406: U3.2 v141.78,62.26 | R14.2 132.25,45.4 135.13,48.28 135.13,51.58 136.74,53.2 IC3.5 139.97,53.22 141.43,53.22 143.75,55.54 143.75,62.23 v143.76,62.25
  Bottom 0.406: v143.76,62.25 v141.79,62.25 v141.78,62.26
IC1_P18  (via drill 0.3)
  Top 0.406: v141.85,60.92 141.85,60.98 141.84,60.99 U3.1 | v144.65,60.92 144.65,55 141.57,51.92 IC3.4 139.86,51.84 137.41,51.84 136.14,50.57 136.14,47.27 134.44,45.56 R13.2
  Bottom 0.406: v141.85,60.92 v144.65,60.92
IC1_P19  (via drill 0.3)
  Top 0.406: U3.3 141.93,63.53 142.85,62.61 v142.85,58.95 142.85,56.29 140.98,54.42 140,54.42 IC3.6 | R15.2 137.23,46.32 137.92,47.01 v144.53,47.01
  Bottom 0.406: v144.53,47.01 144.53,57.15 142.85,58.83 v142.85,58.95
IC1_P20  (via drill 0.3)
  Top 0.406: U3.4 138.56,64.8 136.1,62.33 136.1,57.34 137.72,55.72 139.94,55.72 IC3.7 141.06,55.74 v141.99,56.66 | v142.75,46 140.99,46 140.65,45.66 R16.2
  Bottom 0.406: v141.99,56.66 141.99,51.33 142.75,50.57 v142.75,46
IC1_P21
  Top 0.406: IC3.9 130.75,57.87 | 130.75,57.87 133.1,60.22 133.1,64.82 134.3,66.02 140.01,66.02 U3.5 | R17.2 129.09,59.54 130.75,57.87
IC1_P22  (via drill 0.3)
  Top 0.406: v133.1,58.22 133.1,56.42 132.42,55.74 IC3.10 129.25,55.74 R18.2 | v134.3,67.32 140.04,67.32 U3.6
  Bottom 0.406: v133.1,58.22 133.1,66.12 v134.3,67.32
IC1_P23  (via drill 0.3)
  Top 0.406: v134.1,64.12 134.1,55.82 132.75,54.47 IC3.11 128.08,54.47 R19.2 | v135.8,68.52 139.97,68.52 U3.7
  Bottom 0.406: v134.1,64.12 134.1,64.52 135.8,66.22 v135.8,68.52
IC1_P24  (via drill 0.3)
  Top 0.406: U3.8 137.25,69.88 v137.2,69.82 | v135,62.92 135,54.62 133.5,53.12 130.83,53.12 IC3.12 129.63,53.2 128.52,52.09 R20.2
  Bottom 0.406: v137.2,69.82 137.2,65.12 v135,62.92
IC1_P25  (via drill 0.3)
  Top 0.406: R22.2 88.83,31.85 90.42,30.25 91.75,30.25 IC4.5 93.71,30.26 v93.73,30.25 | U4.2 91.67,22.63 v89.66,22.63
  Bottom 0.406: v93.73,30.25 89.66,26.18 v89.66,22.63
IC1_P26
  Top 0.406: U4.1 91.81,23.9 93.22,23.9 94.74,25.42 94.74,30.5 93.71,31.53 IC4.4 91.75,31.52 90.68,31.52 89.99,32.2 89.99,32.74 R21.2
IC1_P27  (via drill 0.3)
  Top 0.406: R23.2 88.67,29.21 88.9,28.98 91.75,28.98 IC4.6 93.71,28.99 v93.73,28.98 | v93.73,21.36 91.81,21.36 U4.3
  Bottom 0.406: v93.73,28.98 92.71,27.96 92.71,22.37 v93.73,21.36
IC1_P28  (via drill 0.3)
  Top 0.406: IC4.7 91.75,27.71 90.93,27.71 89.81,26.58 R24.2 88.42,24.69 v88.39,24.66 | U4.4 89.99,20.02 v89.92,20.09
  Bottom 0.406: v89.92,20.09 88.39,21.61 v88.39,24.66
IC1_P29  (via drill 0.3)
  Top 0.406: v97.79,26.44 97.8,26.45 IC4.9 100.98,26.44 101.6,26.44 103.69,24.35 R25.2 | v89.92,18.82 91.67,18.82 U4.5
  Bottom 0.406: v97.79,26.44 97.79,22.88 93.73,18.82 v89.92,18.82
IC1_P30  (via drill 0.3)
  Top 0.406: U4.6 89.99,17.48 v89.92,17.55 | v99.06,27.71 100.95,27.71 IC4.10 103.17,27.72 R26.2
  Bottom 0.406: v89.92,17.55 93.98,17.55 99.06,22.63 v99.06,27.71
IC1_P31  (via drill 0.3)
  Top 0.406: v99.06,28.98 99.07,28.99 IC4.11 103.55,28.99 R27.2 | v95.25,24.41 95.25,21.1 93.47,19.33 93.47,16.79 92.96,16.28 91.81,16.28 U4.7
  Bottom 0.406: v99.06,28.98 98.55,28.98 95.25,25.68 v95.25,24.41
IC1_P32
  Top 0.406: U4.8 92.89,14.94 94.11,16.15 94.11,18.69 96.27,20.85 96.27,28.22 98.3,30.25 100.95,30.25 IC4.12 102.12,30.26 103.63,31.77 103.84,31.77 R28.2
IC1_P33  (via drill 0.3)
  Top 0.406: v108.2,30.25 110.21,30.25 IC5.5 111.77,30.26 112.01,30.5 v112.01,31.52 | U5.2 108.53,22.56 v108.51,22.58
  Bottom 0.406: v108.2,30.25 108.2,22.88 v108.51,22.58 | R30.2 112.66,33.18 112.01,32.53 v112.01,31.52
IC1_P34  (via drill 0.3)
  Top 0.406: v108.2,31.52 110.21,31.52 IC5.4 111.01,31.53 112.01,32.53 v112.01,33.55 | U5.1 110.3,24.34 v109.73,24.91
  Bottom 0.406: v109.73,24.91 109.35,25.3 109.35,30.38 v108.2,31.52 | v112.01,33.55 112.01,34.05 R29.2
IC1_P35  (via drill 0.3)
  Top 0.406: U5.3 108.53,21.29 107.44,22.37 107.44,27.45 108.97,28.98 110.21,28.98 IC5.6 111.93,28.99 v111.94,29
  Bottom 0.406: v111.94,29 111.94,29.42 R31.2
IC1_P36  (via drill 0.3)
  Top 0.406: U5.4 111.18,20.02 112.27,21.1 v112.27,27.2 111.76,27.71 110.24,27.71 IC5.7
  Bottom 0.406: R32.2 113.44,28.37 v112.27,27.2
IC1_P37  (via drill 0.3)
  Top 0.406: v119.38,25.17 119.41,25.17 119.42,25.18 IC5.9 121.61,24.27 R33.2 | v108.46,18.82 110.23,18.82 U5.5
  Bottom 0.406: v119.38,25.17 113.03,18.82 v108.46,18.82
IC1_P38  (via drill 0.3)
  Top 0.406: U5.6 111.44,17.48 112.01,18.06 112.01,19.58 v113.54,21.1 | v121.16,27.71 121.14,27.72 IC5.10 119.44,27.71 120.65,27.71 121.6,26.76 R34.2
  Bottom 0.406: v121.16,27.71 120.14,27.71 v113.54,21.1
IC1_P39  (via drill 0.3)
  Top 0.406: U5.7 111.44,16.21 112.67,17.45 112.67,18.97 114.55,20.85 v114.55,23.39 | v121.08,29.23 120.83,28.98 | 120.83,28.98 119.44,28.98 IC5.11 | R35.2 121.15,29.23 120.9,28.98 120.83,28.98
  Bottom 0.406: v114.55,23.39 120.4,29.23 v121.08,29.23
IC1_P40
  Top 0.406: U5.8 111.44,14.94 113.28,16.79 113.28,18.31 115.32,20.34 115.32,27.45 118.11,30.25 119.41,30.25 IC5.12 120.66,30.26 122.17,31.77 123.19,31.77 123.44,31.52 123.04,31.52 R44.2
IC6_P0
  Top 0.406: U6.1 130.7,23.53 133.35,26.18 133.35,29.99 132.46,30.88 | 132.46,30.88 132.33,31.01 130.74,31.01 IC6.4 | R45.2 137.24,35.66 132.46,30.88
IC6_P1  (via drill 0.3)
  Top 0.406: U6.2 128.34,22.05 v128.27,22.12 | IC6.5 130.72,29.74 v128.02,29.74 128.02,37.45 128.86,38.29 R46.2
  Bottom 0.406: v128.02,29.74 127,28.72 127,23.39 v128.27,22.12
IC6_P2  (via drill 0.3)
  Top 0.406: IC6.6 128.03,28.48 | U6.3 130.51,20.6 128.02,20.6 127,21.61 127,27.45 128.03,28.48 | R47.2 131.65,36.93 v131.57,36.85 | v127,31.01 127,29.51 128.03,28.48
  Bottom 0.406: v131.57,36.85 129.29,36.85 127,34.57 v127,31.01
IC6_P3  (via drill 0.3)
  Top 0.406: U6.4 131.75,19.51 133.35,21.1 v133.35,25.17 | v128.78,27.2 130.72,27.2 IC6.7 | R48.2 134.44,37.18 v134.37,37.11
  Bottom 0.406: v133.35,25.17 133.35,25.42 131.57,27.2 | 131.57,27.2 v128.78,27.2 | v134.37,37.11 134.37,29.99 131.57,27.2
IC6_P4  (via drill 0.3)
  Top 0.406: v137.92,25.93 137.94,25.94 IC6.9 141.48,24.41 141.48,21.36 142.57,20.27 R49.2 | v128.78,18.31 130.62,18.31 U6.5
  Bottom 0.406: v137.92,25.93 130.3,18.31 v128.78,18.31
IC6_P5  (via drill 0.3)
  Top 0.406: v137.92,27.2 137.94,27.21 IC6.10 140.96,27.21 142.24,25.93 142.24,23.39 143.08,22.55 R50.2 | v127.51,16.79 130.51,16.79 U6.6
  Bottom 0.406: v137.92,27.2 136.65,27.2 127.51,18.06 v127.51,16.79
IC6_P6  (via drill 0.3)
  Top 0.406: U6.7 131.75,15.7 132.59,16.53 132.59,19.07 134.37,20.85 v134.37,26.18 | v137.92,28.47 137.94,28.48 IC6.11 139.94,28.47 141.22,28.47 144.03,25.67 R51.2
  Bottom 0.406: v134.37,26.18 136.65,28.47 v137.92,28.47
IC6_P7  (via drill 0.3)
  Top 0.406: U6.8 131.75,14.43 133.6,16.28 133.6,18.82 135.64,20.85 135.64,27.45 137.92,29.74 139.92,29.74 IC6.12 141.97,29.75 v141.99,29.74 | R52.2 140.66,36.91 v140.72,36.85
  Bottom 0.406: v140.72,36.85 140.72,34.82 142.75,32.79 142.75,30.5 v141.99,29.74
ID_SC
  Bottom 0.406: JP1.32 82.27,56.89 81.03,55.65 78.49,55.65 77.72,54.89 77.72,53.36 75.69,51.33 75.69,44.48 JP4.27
ID_SD
  Bottom 0.406: JP1.30 82.27,54.35 81.03,53.11 78.99,53.11 76.45,50.57 76.45,43.2 74.17,40.92 72.18,40.92 JP4.28
MISO
  Bottom 0.406: JP4.22 71.07,34.59 71.07,34.36 72.14,33.3 75.77,33.3 76.17,32.89 81.03,32.89 JP1.14
MOSI
  Top 0.406: JP1.12 82.27,31.62 81,32.89 77.72,32.89 75.59,30.76 72.39,30.76 71.09,32.05 JP4.20
N$1
  Top 0.254: 38.35,23.93 IC7.7
  Top 0.406: R53.1 42.42,29.49 38.35,25.42 38.35,23.93
N$2
  Top 0.406: IC7.8 37,26.1 38.61,27.71 R54.1
N$12  (via drill 0.3)
  Top 0.406: IC102.3 105.62,40.37 106.68,41.42 v106.93,41.42 | BAT.+ 147.25,33.62 144.27,36.6 144.27,40.15 v142.24,42.19
  Bottom 0.406: v142.24,42.19 127.76,42.19 122.94,37.36 109.98,37.36 106.93,40.41 v106.93,41.42
N$27
  Top 0.406: Q101.1 99.05,41.28 103.66,41.28 104.25,40.69 104.25,39.27 104.27,39.26 IC102.2
N$29
  Top 0.406: Q101.2 102.59,38.76 IC102.1
N$35
  Top 0.254: 60.65,53.52 C12.2
  Top 0.406: IC13.1 58.8,54.13 59.4,53.52 60.65,53.52
N$36
  Top 0.406: IC13.4 58.57,57.94 60.15,59.52 C13.2
N$39
  Top 0.254: 54.66,55.42 55.65,55.42 IC13.2
  Top 0.406: C14.1 54.05,50.35 53.61,50.79 53.61,54.37 54.66,55.42
N$43
  Top 0.254: 55.62,60.42 IC13.6
  Top 0.406: C15.2 54.05,67.16 53.65,66.76 53.65,61.22 54.45,60.42 55.62,60.42
N$44  (via drill 0.6)
  Top 0.61: 6.26,69.55 R10.2 v9.93,69.16
  Top 0.813: Q1.G 6.26,69.55
  Bottom 0.61: v9.93,69.16 14.95,69.16 D9.A
N$52
  Top 0.406: IC13.3 60.51,56.67 C12.1
N$54
  Top 0.254: IC13.5 56.68,59.21 | 60.8,62.42 C13.1
  Top 0.406: 56.68,59.21 59.89,62.42 60.8,62.42
ONEWIRE  (via drill 0.3)
  Top 0.254: 15.31,16.53 R3.1
  Top 0.305: R3.1 15.5,17.41 | 38.31,17.66 IC7.2 | 27.94,18.62 29.97,18.62
  Top 0.406: 15.5,17.41 16.72,18.62 27.94,18.62 26.42,20.15 26.42,25.42 29.21,28.22 v35.05,28.22 | 38.31,17.66 38.31,18.82 37.8,19.33 33.78,19.33 33.08,18.62 29.97,18.62 31.18,19.83 Q2.2 | JP1.11 78.81,31.59 75.44,28.22 v42.52,28.22 | J103.4 10.03,12.08 14.48,16.53 15.31,16.53
  Bottom 0.406: v42.52,28.22 v35.05,28.22
PCTLZ
  Top 0.254: 39.51,23.88 IC7.6 | Q2.1 30.3,21.61 32.26,21.61 33.02,20.85 | 33.68,20.85 R55.2
  Top 0.406: 39.51,23.88 39.51,22.52 37.95,20.95 R55.2 | 33.02,20.85 33.68,20.85
Q1_P0  (via drill 0.3)
  Top 0.406: P13.1 80.35,81.27 82.15,79.47 82.15,77.27 86.33,73.09 86.33,66.16 v86.35,66.14 | v86.35,63.23 88.16,61.42 91.43,61.42 U1.18
  Bottom 0.406: v86.35,66.14 v86.35,63.23
Q1_P1
  Top 0.406: P13.3 83.85,81.27 85.5,79.62 85.5,77.36 88.04,74.82 88.04,64.35 89.76,62.62 91.4,62.62 U1.17
Q1_P2  (via drill 0.3)
  Top 0.406: P13.2 80.32,77.77 85.35,72.74 85.35,65.74 87.17,63.92 v87.3,63.92 | v89.6,63.92 91.43,63.92 U1.16
  Bottom 0.406: v87.3,63.92 v89.6,63.92
Q1_P3  (via drill 0.3)
  Top 0.406: P13.4 83.75,77.63 87.25,74.13 v87.25,65.22 | v89.61,65.21 U1.15
  Bottom 0.406: v87.25,65.22 v89.6,65.22 v89.61,65.21
Q1_P4
  Top 0.406: P13.7 88.87,79.4 88.87,67.62 90.07,66.42 91.39,66.42 U1.14
Q1_P5
  Top 0.406: P13.9 94.3,81.27 96,79.58 96,71.28 92.44,67.72 91.48,67.72 U1.13
Q1_P6
  Top 0.406: U1.12 90.35,69.02 89.73,69.65 89.73,76.57 90.75,77.59 P13.8
Q1_P7
  Top 0.406: U1.11 92.81,70.29 94.25,71.73 P13.10
Q2_P0
  Top 0.406: U2.18 107.81,61.4 105.9,63.31 105.9,70.11 99.45,76.56 99.45,79.48 P13.13
Q2_P1
  Top 0.406: U2.17 107.9,62.67 106.7,63.88 106.7,70.77 103,74.47 103,79.52 P13.15
Q2_P2  (via drill 0.3)
  Top 0.406: U2.16 107.78,63.94 v107.7,64.03
  Bottom 0.406: P13.14 101.25,70.47 v107.69,64.03 v107.7,64.03
Q2_P3  (via drill 0.25)
  Top 0.406: U2.15 107.86,65.21 v107.8,65.27
  Bottom 0.406: v107.8,65.27 104.75,68.32 P13.16
Q2_P4  (via drill 0.25)
  Top 0.406: v107.8,66.61 109.53,66.61 109.62,66.52 109.74,66.52 U2.14
  Bottom 0.406: P14.1 117.75,81.2 114.8,78.25 114.8,75.94 107.8,68.94 v107.8,66.61
Q2_P5
  Top 0.406: P14.3 121.35,81.26 123.1,79.51 123.1,77.02 120.49,74.41 118.28,74.41 111.61,67.75 U2.13
Q2_P6
  Top 0.406: P14.2 117.75,75.29 111.48,69.02 U2.12
Q2_P7  (via drill 0.3)
  Top 0.406: v111.46,70.3 U2.11
  Bottom 0.406: P14.4 113.79,70.3 v111.46,70.3
Q3_P0
  Top 0.406: U3.18 128.57,60.99 125.7,63.85 125.7,75.91 126.5,76.71 126.5,79.51 P14.7
Q3_P1  (via drill 0.25)
  Top 0.406: U3.17 130.68,62.22 v128.78,62.22
  Bottom 0.406: v128.78,62.22 128.68,62.22 126.3,64.6 126.3,72.61 129.9,76.21 129.9,79.41 P14.9
Q3_P2
  Top 0.406: U3.16 128.62,63.53 126.81,65.34 126.81,75.11 128.17,76.48 128.17,77.69 P14.8
Q3_P3
  Top 0.406: P14.10 131.75,76.26 127.66,72.18 127.66,65.98 128.92,64.72 130.64,64.72 U3.15
Q3_P4  (via drill 0.25, 0.3)
  Top 0.406: P14.13 138.85,81.26 140.25,79.87 140.25,76.71 134.49,70.95 v134.43,71.01 | v128.71,66.12 130.66,66.12 U3.14
  Bottom 0.406: v134.43,71.01 134.43,71 132,68.57 132,66.42 131.7,66.12 v128.71,66.12
Q3_P5
  Top 0.406: P14.15 142.35,81.26 143.85,79.77 143.85,77.11 141.39,74.66 140.13,74.66 132.8,67.32 130.73,67.32 U3.13
Q3_P6
  Top 0.406: P14.14 133.1,72.11 133.1,69.82 131.9,68.62 130.73,68.62 U3.12
Q3_P7  (via drill 0.3)
  Top 0.406: v128.91,69.82 130.66,69.82 U3.11
  Bottom 0.406: P14.16 142.25,77.56 140.49,75.81 136.8,75.81 130.81,69.82 v128.91,69.82
Q4_P0
  Top 0.406: P15.20 80.4,8.27 81.75,9.62 83.62,9.62 86.21,12.21 92.46,12.21 94.74,14.5 94.74,18.31 100.26,23.83 U4.18
Q4_P1
  Top 0.406: P15.18 86.8,11.33 92.58,11.33 95.5,14.25 95.5,18.06 100,22.56 U4.17
Q4_P2
  Top 0.406: U4.16 100.26,21.29 96.27,17.29 96.27,13.99 92.84,10.56 87.5,10.56 85.6,8.66 85.6,7.64 84.58,6.63 82.1,6.63 P15.19
Q4_P3  (via drill 0.3)
  Top 0.406: v95,11.45 97.03,13.48 97.03,16.79 100.08,19.83 100.91,19.83 U4.15
  Bottom 0.406: P15.17 85.6,6.63 88.14,6.63 89.05,7.54 89.05,8.81 91.69,11.45 v95,11.45
Q4_P4
  Top 0.406: U4.14 100,18.75 98.04,16.79 98.04,13.23 94.74,9.93 92.41,9.93 P15.14
Q4_P5
  Top 0.406: U4.13 101.02,17.55 100.08,17.55 98.81,16.28 98.81,12.83 P15.12
Q4_P6  (via drill 0.3)
  Top 0.406: v103.38,16.28 101.16,16.28 U4.12
  Bottom 0.406: P15.13 92.6,6.63 94.74,6.63 96.01,7.9 96.01,9.93 96.77,10.69 101.35,10.69 103.38,12.72 v103.38,16.28
Q4_P7
  Top 0.406: P15.11 94.41,4.77 96.01,6.37 96.01,8.4 99.57,11.96 99.57,14.5 100,14.94 U4.11
Q5_P0
  Top 0.406: U5.18 118.55,23.83 116.33,21.61 116.33,20.34 113.92,17.93 113.92,14.88 111.51,12.47 105.45,12.47 P15.8
Q5_P1
  Top 0.406: U5.17 119.58,22.63 118.62,22.63 117.09,21.1 117.09,19.83 114.55,17.29 114.55,14.25 112.01,11.71 107.19,11.71 104.77,9.29 104.77,8.27 P15.6
Q5_P2
  Top 0.406: U5.16 118.55,21.29 117.86,20.6 117.86,19.33 115.32,16.79 115.32,13.48 112.78,10.94 108.71,10.94 106.68,8.91 106.68,7.9 105.41,6.63 103.1,6.63 P15.7
Q5_P3  (via drill 0.3)
  Top 0.406: v121.67,20.09 119.72,20.09 U5.15 | v109.98,6.63 109.98,8.91 111.25,10.18 113.28,10.18 v115.06,11.96
  Bottom 0.406: P15.5 104.83,4.77 106.68,6.63 v109.98,6.63 | v115.06,11.96 115.06,13.38 121.67,19.99 v121.67,20.09
Q5_P4
  Top 0.406: U5.14 118.55,18.75 116.33,16.53 116.33,9.69 P16.20
Q5_P5  (via drill 0.3)
  Top 0.406: U5.13 121.34,17.48 v121.41,17.55
  Bottom 0.254: 120.14,9.38 P16.18
  Bottom 0.406: v121.41,17.55 120.14,16.28 120.14,9.38
Q5_P6
  Top 0.254: 119.38,6.4 P16.19
  Top 0.406: U5.12 119.13,16.21 119.06,16.28 118.62,16.28 117.35,15.01 117.35,11.71 119.38,9.67 119.38,6.4
Q5_P7
  Top 0.406: U5.11 121.17,14.94 123.19,12.92 123.19,6.71 P16.17
Q6_P0
  Top 0.254: P16.14 128.25,8.89
  Top 0.406: 128.25,8.89 130.81,11.45 131.83,11.45 134.37,13.99 134.37,18.31 136.65,20.6 136.65,21.87 138.18,23.39 139.97,23.39 U6.18
Q6_P1  (via drill 0.3)
  Top 0.406: U6.17 138.25,22.05 v138.18,22.12
  Bottom 0.406: v138.18,22.12 134.62,18.56 134.62,11.14 P16.12
Q6_P2
  Top 0.406: U6.16 138.1,20.78 135.38,18.06 135.38,13.74 132.08,10.44 131.06,10.44 130.05,9.42 130.05,6.57 P16.13
Q6_P3
  Top 0.406: U6.15 138.36,19.51 136.14,17.29 136.14,12.47 133.6,9.93 133.6,6.63 P16.11
Q6_P4
  Top 0.406: U6.14 138.36,18.24 136.91,16.79 136.91,10.12 P16.8
Q6_P5  (via drill 0.3)
  Top 0.406: v142.24,17.04 140.12,17.04 U6.13
  Bottom 0.406: P16.6 142.76,8.78 142.76,16.52 v142.24,17.04
Q6_P6  (via drill 0.3)
  Top 0.406: P16.7 138.86,4.77 140.46,6.37 v140.46,9.42 | v138.43,15.64 139.99,15.64 U6.12
  Bottom 0.406: v140.46,9.42 141.73,10.69 141.73,13.48 139.57,15.64 v138.43,15.64
Q6_P7
  Top 0.406: P16.5 142.25,4.86 144.02,6.63 144.02,11.58 141.1,14.5 140.12,14.5 U6.11
RX
  Top 0.254: IC13.8 56.79,63.02 57.9,64.13 57.9,65.24 61.77,69.11 74.86,69.11 76.35,70.61 76.35,81.31 78.9,83.85 149.34,83.85 153.16,80.03
  Top 0.406: 153.16,80.03 153.16,58.83 RS232.3
RXD  (via drill 0.25, 0.3)
  Top 0.254: JP4.9 73.42,19.4 | IC13.9
  Top 0.406: 73.42,19.4 72.25,20.57 55.96,20.57 v51.38,25.15 | v46.6,63.02 IC13.9
  Bottom 0.254: v51.38,25.15 51.31,25.15 | JP1.7 79.73,26.67 77.22,24.15 77.22,23.09 | 73.48,19.35 JP4.9
  Bottom 0.406: v46.6,63.02 46.3,62.72 46.3,60.4 49.28,57.43 49.28,44.47 51.31,42.44 51.31,25.15 | 77.22,23.09 73.48,19.35
SCLK
  Bottom 0.406: JP4.24 70.88,37.09 72.14,35.84 75.62,35.84 76.07,35.38 80.98,35.38 JP1.16
TX  (via drill 0.3)
  Top 0.254: IC13.7 55.7,61.72 57.05,61.72 59.18,63.86 v59.18,65.3
  Bottom 0.254: 153.16,80.04 149.35,83.85 78.9,83.85 76.35,81.31 76.35,70.61 74.86,69.11 63,69.11 v59.18,65.3
  Bottom 0.406: RS232.2 151.57,53.04 153.16,54.63 153.16,80.04
TXD  (via drill 0.3)
  Top 0.254: JP4.7 73.31,16.81
  Top 0.406: IC13.10 47.52,61.75 v47.4,61.62 | 73.31,16.81 72,18.12 | 72,18.12 54.12,18.12 v52.21,20.03 | 72,18.12 75,18.12 77.22,20.34 77.22,26.54 JP1.9
  Bottom 0.254: v52.21,20.03 52.32,20.14
  Bottom 0.406: v47.4,61.62 50.19,58.83 50.19,46.09 52.32,43.96 52.32,20.14
VIN-ONEWIRE  (via drill 0.6)
  Top 0.406: J103.2 12.07,11.88 13.76,13.57 16.67,13.57 18.3,15.2 R3.2
  Top 0.61: v20.6,16.72 R3.2
  Bottom 0.813: OW.2 17.88,23.12 20.6,20.4 v20.6,16.72
VIN_RELAIS  (via drill 0.3, 0.35, 0.6)
  Top 0.406: P13.17 P13.18 108.2,77.72 108.2,73.14 U2.10 | P13.5 P13.6 | P13.11 P13.12 | P15.15 P15.16 | P14.12 135.25,76.56 130.7,72.01 130.7,71.16 U3.10 | U1.10 91.54,71.56 v92.69,72.71 | v121.16,11.96 119.65,13.47 U5.10 | U4.10 101.09,11.61 P15.10 | v138.43,13.1 139.99,13.1 U6.10
  Top 0.61: P14.11 135.2,81.31 135.2,82.05 135.25,82 | 124.8,82.25 124.8,82.15 | 124.8,81.31 P14.5 124.75,82.1 124.8,82.15 | 124.8,82.15 124.7,82.15 | P13.17 108.25,82.1 108.3,82.15 108.2,82.15 | 97.75,82.1 97.8,82.15 | 87.25,4.09 87.25,3.57 | 97.7,3.32 97.7,3.52 | 97.7,4.72 P15.9 97.75,3.57 97.7,3.52 | 97.7,3.52 98,3.52 | 108.3,4.72 P15.3 108.25,3.47 108.3,3.42 108.3,3.32 | 124.7,4.72 P16.15 124.75,3.47 | 135.2,4.72 P16.9 135.25,3.47 | 145.7,4.72 P16.3 | 87.25,81.95 87.25,82.19
  Top 0.813: P16.4 P16.3 145.88,4.77 147.63,6.52 150.27,6.52 152.93,9.19 JP2.2 | P14.18 P14.17 145.75,82.06 144.75,83.05 136.2,83.05 135.2,82.05 134.2,83.05 125.6,83.05 124.8,82.25 | 135.25,82 P14.11 P14.12 | 124.8,82.15 124.8,81.31 | 124.7,82.15 123.8,83.05 109.2,83.05 108.3,82.15 | 108.2,82.15 107.4,82.95 98.6,82.95 97.8,82.15 97,82.95 88.25,82.95 87.25,81.95 P13.5 | P13.11 97.75,82.1 | P14.5 P14.6 | P15.15 87.25,4.09 86.23,3.07 78.49,3.07 76.71,1.29 63.5,1.29 v60.71,4.09 | 87.25,3.57 88.1,2.72 97.1,2.72 97.7,3.32 | 97.7,3.52 97.7,4.72 | 98,3.52 98.8,2.72 107.6,2.72 108.3,3.42 108.3,4.72 | P15.9 P15.10 | 108.3,3.32 109,2.62 124,2.62 124.7,3.32 124.7,4.72 | 124.75,3.47 125.6,2.62 134.5,2.62 135.2,3.32 135.2,4.72 | 135.25,3.47 136.1,2.62 145,2.62 145.7,3.32 145.7,4.72 | P16.15 P16.16 | P16.9 P16.10 | P15.3 P15.4 | v58.42,12.04 v58.42,16.53 | v62.99,53.12 62.99,64.28 67.06,68.35 75.44,68.35 77.22,70.13 77.22,80.79 79.5,83.08 86.36,83.08 87.25,82.19
  Bottom 0.254: 124.71,8.4 124.71,8.31 | v62.99,53.12 62.99,52.87
  Bottom 0.406: v92.69,72.71 92.83,72.71 97.75,77.63 P13.12 | 124.71,8.4 v121.16,11.96 | 124.71,8.31 P16.16 | P16.10 135.25,9.92 v138.43,13.1
  Bottom 0.813: v58.42,12.04 58.42,6.37 v60.71,4.09 | v58.42,16.53 58.42,48.3 62.99,52.87

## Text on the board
Top: Top | Output Board / 2019 - V1.0
Bottom: Bot
tDocu: 1: +12V / 2: TX / 3: RX / 4: Gnd | +5V | +3.3V | Gnd | One Wire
